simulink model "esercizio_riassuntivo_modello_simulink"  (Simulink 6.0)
settings: Solver=ode45  StartTime=0.0  StopTime=T  RelTol=1e-3
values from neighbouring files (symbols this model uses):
  Tc = 0.01    [createsimulation.m]    (also in esercizio_riassuntivo_script1.m = 0.1)

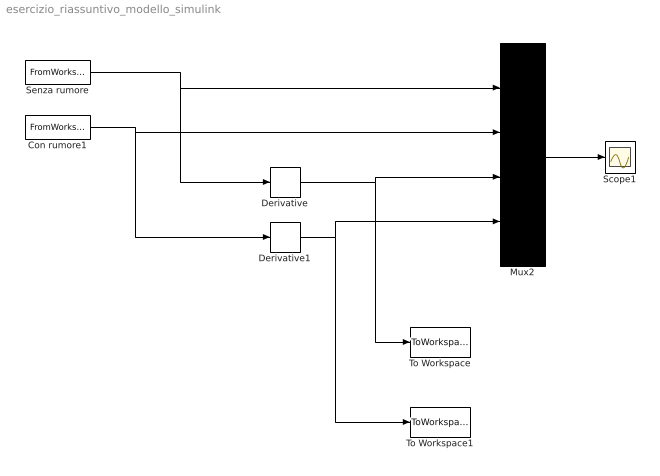
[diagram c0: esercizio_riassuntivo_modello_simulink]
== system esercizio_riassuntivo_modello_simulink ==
  Con rumore1 : FromWorkspace  VariableName=[t z]  SampleTime=Tc
  Derivative : Derivative
  Derivative1 : Derivative
  Mux2 : Mux
  Scope1 : Scope
  Senza rumore : FromWorkspace  VariableName=[t y]  SampleTime=Tc
  To Workspace : ToWorkspace  VariableName=dy  SampleTime=Tc  SaveFormat=Array
  To Workspace1 : ToWorkspace  VariableName=dz  SampleTime=Tc  SaveFormat=Array
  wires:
  Mux2/1 -> Scope1/1
  Senza rumore/1 -> Mux2/1, Derivative/1
  Con rumore1/1 -> Mux2/2, Derivative1/1
  Derivative/1 -> Mux2/3, To Workspace/1
  Derivative1/1 -> Mux2/4, To Workspace1/1
